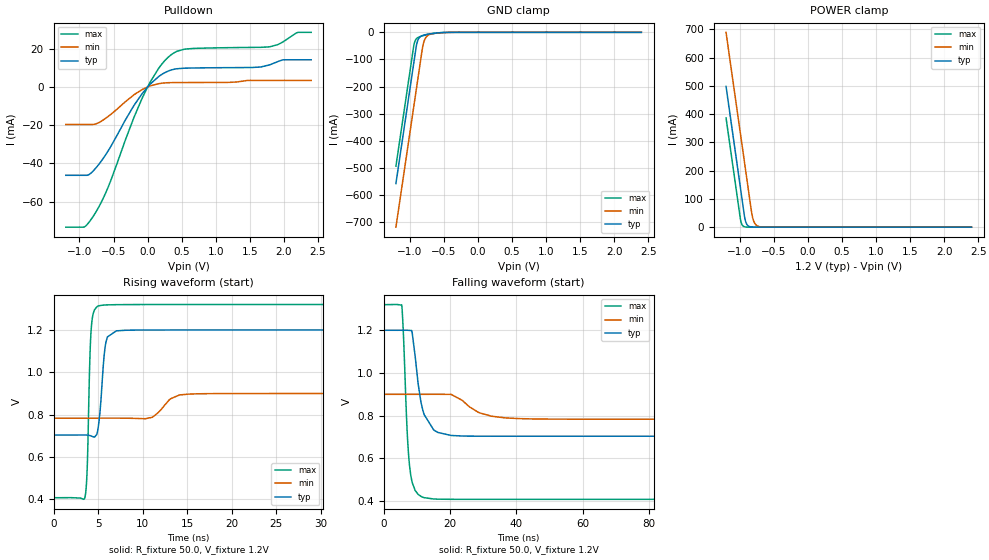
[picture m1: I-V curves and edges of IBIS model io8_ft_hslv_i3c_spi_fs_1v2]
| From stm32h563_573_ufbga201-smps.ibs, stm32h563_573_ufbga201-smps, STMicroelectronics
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[Model]   io8_ft_hslv_i3c_spi_fs_1v2
Model_type I/O_open_drain
Polarity   Non-Inverting
Enable   Active-Low
| CAP_THRESHOLD on pad IOFT is "UDTCAPC" :
| Rising=20.0% of vddiom   Falling=80.0% of vddiom
| C_comp min and max val. don't necessarily correlate with the min and max pvt
| but are the smallest and greatest pad capacitance found.
| var   typ   min   max
C_comp   3.41805pF  3.40000pF  3.42900pF
|C_comp_pulldown   3.41805pF  3.40000pF  3.42900pF
Vinl = 450.0mV
Vinh = 660.0mV
Vmeas = 600.0mV   | Reference voltage for timing measurements
Cref  = 50.0pF   | Timing specification test load capacitance value
Rref  = 1.0MOhm   | Timing specification test load resistance value
Vref  = 660.0mV   | Timing specification test load voltage
[Model Spec]
| TIME_THRESHOLD on pin ZII2CV11 is "CMOS" :
| Rising=40.0% of vdd   Falling=60.0% of vdd
Vinl 447.80000mV 344.80000mV 489.80000mV
Vinh 733.20000mV 535.20000mV 813.20000mV
| variable   typ   min   max
[Temperature Range] 25.0 125.0 -40.0
| variable   typ   min   max
[Voltage Range] 1.2V 900.0mV 1.32V
| variable   typ   min   max
[POWER Clamp Reference] 1.2V 900.0mV 1.32V
| variable   typ   min   max
[GND Clamp Reference] 0V 0V 0V
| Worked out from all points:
|   slope of the pulldown table from 0 to 0.18 V, typ, clamps not added: 30.6 ohm
|   GND clamp passes 1 mA (typ) near -0.52 V on its own axis
|   POWER clamp passes 1 mA (typ) near -0.84 V on its own axis
|   rising waveform, R_fixture 50.0, V_fixture 1.2V: 20-80 % time 546ps typ, 1.57ns min, 329ps max; typ from 0.704 V to 1.2 V
|   falling waveform, R_fixture 50.0, V_fixture 1.2V: 20-80 % time 2.98ns typ, 7.28ns min, 1.58ns max; typ from 1.2 V to 0.704 V
[POWER Clamp]
-1.2V     497.8mA    689.2mA    386.5mA
-990mV    140.8mA    332.2mA    29.53mA
-980mV    123.8mA    315.2mA    17.95mA
-960mV    89.81mA    281.2mA    6.634mA
-930mV    38.81mA    230.2mA    1.49mA
-900mV    12.07mA    179.2mA    334.8uA
-870mV    3.756mA    128.2mA    75.22uA
-820mV    536.4uA    44.98mA    6.246uA
-790mV    166.9uA    18.76mA    1.403uA
-750mV    35.18uA    5.846mA    191.8nA
-590mV    70.09nA    55uA       165.5pA
2.4V      0A         0A         0A
[GND Clamp]
-1.2V     -558.2mA   -719mA     -494.1mA
-940mV    -116.2mA   -277mA     -52.06mA
-930mV    -99.19mA   -260mA     -39.94mA
-900mV    -49.1mA    -209mA     -23.76mA
-880mV    -30.14mA   -175mA     -19.6mA
-850mV    -17.82mA   -124mA     -16.09mA
-810mV    -11.73mA   -56.78mA   -12.91mA
-780mV    -9.444mA   -28.21mA   -10.92mA
-740mV    -7.291mA   -13.16mA   -8.574mA
-640mV    -3.573mA   -4.171mA   -3.954mA
-380mV    -61.75uA   -230.3uA   -20.32uA
2.4V      3.863nA    718.4nA    150.6pA
| variable   typ   min   max
[Pullup Reference] 1.2V 900.0mV 1.32V
| variable   typ   min   max
[Pulldown Reference] 0V 0V 0V
[Pulldown]
-1.2V     -46.17mA   -19.62mA   -73.27mA
-930mV    -46.17mA   -19.62mA   -73.18mA
-770mV    -42.8mA    -19.41mA   -66.04mA
-570mV    -32.88mA   -15.18mA   -51.58mA
-80mV     -3.488mA   -1.363mA   -5.887mA
160mV     5.368mA    1.686mA    9.621mA
340mV     8.782mA    2.251mA    16.66mA
540mV     9.805mA    2.305mA    19.74mA
1.79V     11.53mA    3.428mA    20.94mA
1.98V     14.11mA    3.428mA    23.43mA
2.2V      14.2mA     3.428mA    28.44mA
2.4V      14.2mA     3.428mA    28.54mA
[Ramp]
dV/dt_r 297.78947mV/545.63477ps 69.89501mV/1.5034ns 547.1275mV/326.7524ps
dV/dt_f 297.80518mV/2.9155ns 69.92305mV/6.73126ns 547.13936mV/1.57676ns
R_load = 50.0
| Removed startup time: 0s 0s 0s  .
| Removed end time: 49.4ns.
[Rising Waveform]
R_fixture   = 50.0
V_fixture   = 1.2V
V_fixture_min = 900.0mV
V_fixture_max = 1.32V
0s        703.7mV    783.5mV    408.1mV
3.55ns    703.9mV    783.5mV    414.4mV
3.8ns     703.4mV    783.5mV    570.9mV
4.05ns    701.6mV    783.5mV    1.024V
4.2ns     699.7mV    783.5mV    1.186V
5ns       735mV      783.5mV    1.312V
5.85ns    1.135V     783.5mV    1.318V
7.05ns    1.196V     783.6mV    1.319V
15.15ns   1.2V       897mV      1.32V
49.4ns    1.2V       900mV      1.32V
| Removed startup time: 0s 0s 0s  .
| Removed end time: 199.4ns.
[Falling Waveform]
R_fixture   = 50.0
V_fixture   = 1.2V
V_fixture_min = 900.0mV
V_fixture_max = 1.32V
0s        1.2V       900mV      1.32V
5.45ns    1.2V       900mV      1.318V
6ns       1.2V       900mV      1.167V
7.05ns    1.2V       900mV      738.5mV
7.8ns     1.199V     900mV      566.9mV
8.6ns     1.189V     900mV      488.2mV
12.2ns    805.2mV    900mV      415.9mV
16.3ns    721.6mV    900.1mV    408.9mV
40.7ns    703.7mV    786.3mV    408.1mV
199.4ns   703.7mV    783.5mV    408.1mV
